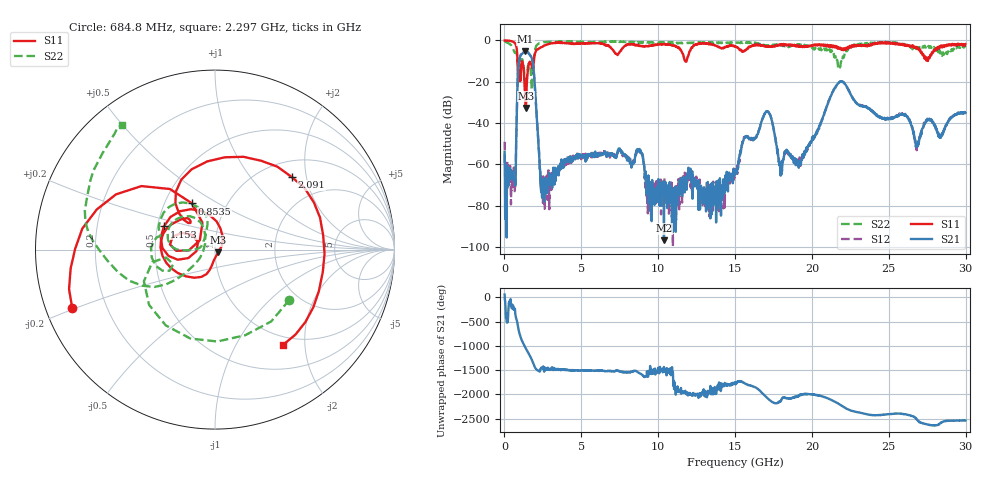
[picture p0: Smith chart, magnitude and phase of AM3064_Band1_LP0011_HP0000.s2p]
# Hz S DB R 50.0
!freq dBS11 angS11 dBS21 angS21 dBS12 angS12 dBS22 angS22
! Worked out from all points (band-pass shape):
!   1600 points, 10 MHz to 29.98 GHz, reference 50 ohm
!   highest |S21| = -5.20 dB at 1.36 GHz (marker M1); lowest = -96.8 dB at 10.38 GHz (marker M2)
!   |S21| within 3 dB of the highest: 1.004 GHz to 1.753 GHz (749.5 MHz wide, 54.4 % of centre)
!   lowest |S11| = -32.7 dB at 1.397 GHz (marker M3), VSWR 1.05, Z = 51.7 - j1.6 ohm
!   |S11| at or under -10 dB: 848.7 MHz to 1.914 GHz (1.066 GHz wide, 77.1 % of centre); 11.75 GHz to 11.84 GHz (89.7 MHz wide, 0.76 % of centre)
!   |S22| runs from -23.9 to -0.3 dB; largest |S21 - S12| = 0.006
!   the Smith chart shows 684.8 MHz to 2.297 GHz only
!   S11 on the Smith chart (normalised r, x): 684.8 MHz: 0.08, -0.20; 853.5 MHz: 0.69, +0.38; 1.153 GHz: 0.54, +0.16; 2.091 GHz: 1.33, +1.65; 2.297 GHz: 0.87, -1.60
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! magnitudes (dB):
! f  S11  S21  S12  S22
! 10 MHz  0.0  -54.1  -49.1  -0.3
! 684.8 MHz  -1.3  -68.2  -65.9  -6.0
! 853.5 MHz  -10.9  -20.2  -20.1  -11.2
! 1.153 GHz  -10.1  -6.5  -6.4  -9.1
! 1.36 GHz  -29.6  -5.2  -5.2  -21.7
! 1.397 GHz  -32.7  -5.2  -5.2  -22.1
! 1.809 GHz  -13.2  -9.5  -9.5  -20.5
! 2.091 GHz  -4.6  -35.6  -35.6  -2.4
! 2.297 GHz  -3.7  -62.5  -62.8  -1.2
! 2.765 GHz  -2.0  -68.0  -65.5  -0.8
! 5.015 GHz  -1.5  -55.5  -56.4  -0.6
! 8.745 GHz  -2.7  -53.4  -53.0  -1.1
! 10 GHz  -2.0  -67.2  -73.5  -0.9
! 10.38 GHz  -1.9  -96.8  -71.9  -1.0
! 15 GHz  -3.0  -64.2  -63.7  -1.2
! 17.05 GHz  -2.9  -34.5  -34.3  -2.7
! 17.97 GHz  -2.3  -65.5  -62.0  -2.1
! 19.99 GHz  -2.7  -48.7  -48.2  -3.3
! 21.85 GHz  -3.5  -20.1  -19.8  -12.4
! 25 GHz  -1.0  -37.7  -37.5  -1.1
! 26.83 GHz  -4.0  -51.6  -49.7  -3.6
! 29.98 GHz  -1.8  -35.0  -34.8  -3.3
